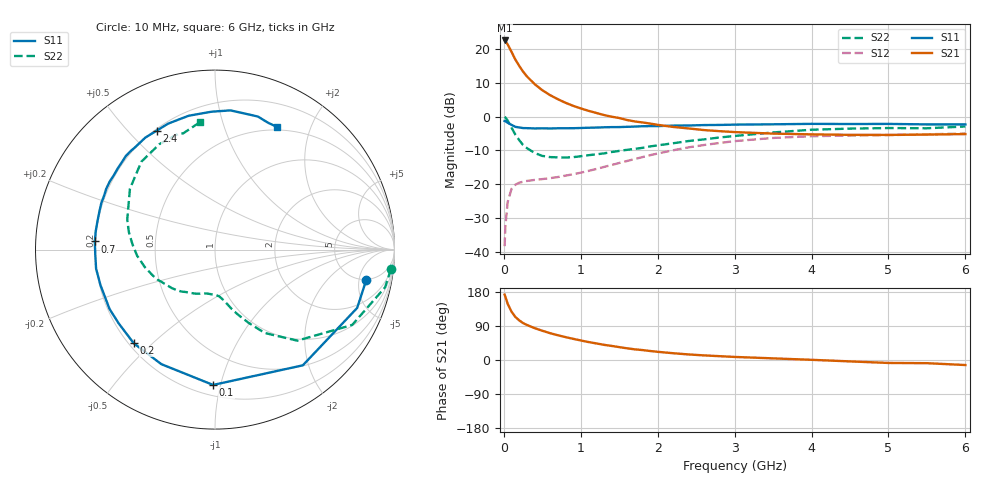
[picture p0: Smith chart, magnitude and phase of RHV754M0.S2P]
! SIEMENS Small Signal Semiconductors
! BFR106
! Si NPN RF Bipolar Junction Transistor in SOT23
! VCE = 0.75 V  IC = 4 mA
! Common Emitter S-Parameters:  August  1996
# GHz  S  MA  R  50
!  f  S11  S21  S12  S22
! GHz  MAG  ANG  MAG  ANG  MAG  ANG  MAG  ANG
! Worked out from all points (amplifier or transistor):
!   36 points, 10 MHz to 6 GHz, reference 50 ohm
!   highest |S21| = 22.5 dB at 10 MHz (marker M1)
!   |S21| within 3 dB of that: start of sweep to 91.77 MHz
!   unconditionally stable (mu >= 1): 626.6 MHz to end of sweep
!   at 250 MHz: K = 0.47, MSG = 16.3 dB, |S12| = -19.2 dB
!   at 1.4 GHz: K = 1.23, MAG = 4.2 dB, |S12| = -14.3 dB
!   at 6 GHz: K = 1.03, MAG = -1.1 dB, |S12| = -5.0 dB
!   S11 on the Smith chart (normalised r, x): 10 MHz: 4.82, -6.31; 100 MHz: 0.27, -0.95; 200 MHz: 0.22, -0.44; 700 MHz: 0.20, +0.03; 2.4 GHz: 0.21, +0.60; 6 GHz: 0.46, +1.52
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0.01  0.8593 -11.5  13.29 172.5  0.0122 85.0  0.9859 -6.3
0.02  0.8562 -22.3  13 166.7  0.024 79.4  0.9708 -12.5
0.05  0.8094 -52.8  11.58 148.2  0.0548 62.9  0.8718 -28.8
0.1  0.7541 -90.8  9.034 127.5  0.0856 46.1  0.6838 -47.9
0.15  0.7048 -115.1  6.93 113.5  0.0985 36.5  0.5408 -59.2
0.2  0.6909 -130.9  5.6 104.6  0.1055 31.9  0.4483 -65.4
0.25  0.676 -142.6  4.61 97.4  0.1091 29.1  0.3805 -70.9
0.3  0.6742 -150.7  3.914 92.5  0.112 28.1  0.3422 -74.4
0.4  0.6681 -162.9  3.018 84.1  0.116 27.7  0.2899 -79.8
0.5  0.6709 -170.9  2.45 77.2  0.1193 29.0  0.2624 -84.6
0.6  0.6677 -177.8  2.076 70.9  0.1233 31.2  0.2522 -89.3
0.7  0.6711 176.1  1.81 65.4  0.1278 33.7  0.2498 -94.4
0.9  0.6734 166.8  1.441 55.9  0.1408 38.8  0.2513 -103.8
1.1  0.6842 157.9  1.216 47.4  0.1576 43.5  0.2687 -114.1
1.3  0.6943 150.8  1.055 40.1  0.1802 46.7  0.2858 -124.1
1.6  0.7057 140.2  0.89 30.9  0.2206 49.0  0.3226 -138.4
2.2  0.7349 121.9  0.703 17.9  0.3175 45.1  0.4034 -166.1
2.4  0.7381 116.2  0.668 14.7  0.3507 42.2  0.4352 -175.5
3.5  0.7685 91.5  0.56 4.3  0.4834 22.5  0.5828 144.4
4.5  0.7759 77.5  0.537 -3.7  0.5248 6.2  0.6639 117.9
5.5  0.7661 67.3  0.542 -8.4  0.5474 -3.2  0.6715 105.3
6  0.7659 63.3  0.551 -13.3  0.562 -9.8  0.7139 96.9
